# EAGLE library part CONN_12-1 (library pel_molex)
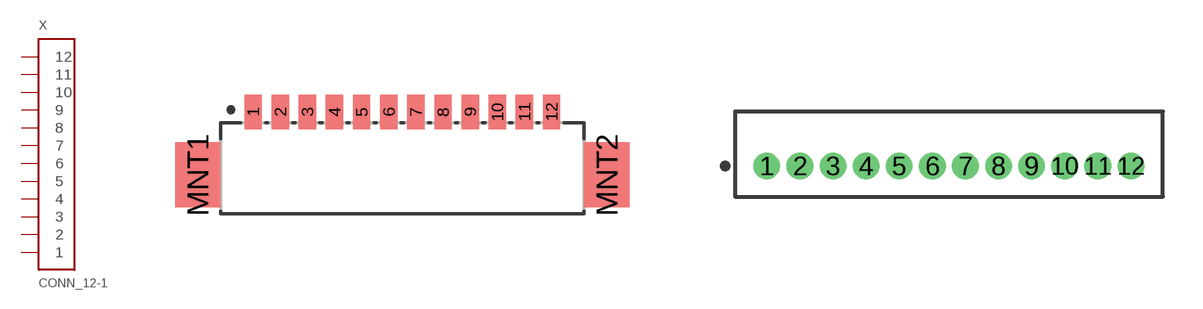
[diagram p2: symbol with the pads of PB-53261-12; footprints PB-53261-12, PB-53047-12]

Designator prefix X

## CONN_12-1-53261  [PB-53261-12]
1  1
2  2
3  3
4  4
5  5
6  6
7  7
8  8
9  9
10  10
11  11
12  12

## CONN_12-1-53047  [PB-53047-12]
Pads as for PB-53261-12

## CONN_12-1-53398  [PB-53398-12]
Pads as for PB-53261-12

## Footprint PB-53261-12 (pad centres in mm)
smd 0.8 x 1.6: 1 -6.875,1.1; 2 -5.625,1.1; 3 -4.375,1.1; 4 -3.125,1.1; 5 -1.875,1.1; 6 -0.625,1.1; 7 0.625,1.1; 8 1.875,1.1; 9 3.125,1.1; 10 4.375,1.1; 11 5.625,1.1; 12 6.875,1.1
smd 2.1 x 3: MNT1 -9.425,-1.8; MNT2 9.425,-1.8

## Footprint PB-53047-12 (pad centres in mm)
drill 0.5: 1 -6.875,0; 2 -5.625,0; 3 -4.375,0; 4 -3.125,0; 5 -1.875,0; 6 -0.625,0; 7 0.625,0; 8 1.875,0; 9 3.125,0; 10 4.375,0; 11 5.625,0; 12 6.875,0

## Footprint PB-53398-12 (pad centres in mm)
smd 0.8 x 1.3: 1 -6.875,1.25; 2 -5.625,1.25; 3 -4.375,1.25; 4 -3.125,1.25; 5 -1.875,1.25; 6 -0.625,1.25; 7 0.625,1.25; 8 1.875,1.25; 9 3.125,1.25; 10 4.375,1.25; 11 5.625,1.25; 12 6.875,1.25
smd 2.1 x 3: PAD1 -9.425,-1.5; PAD2 9.425,-1.5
